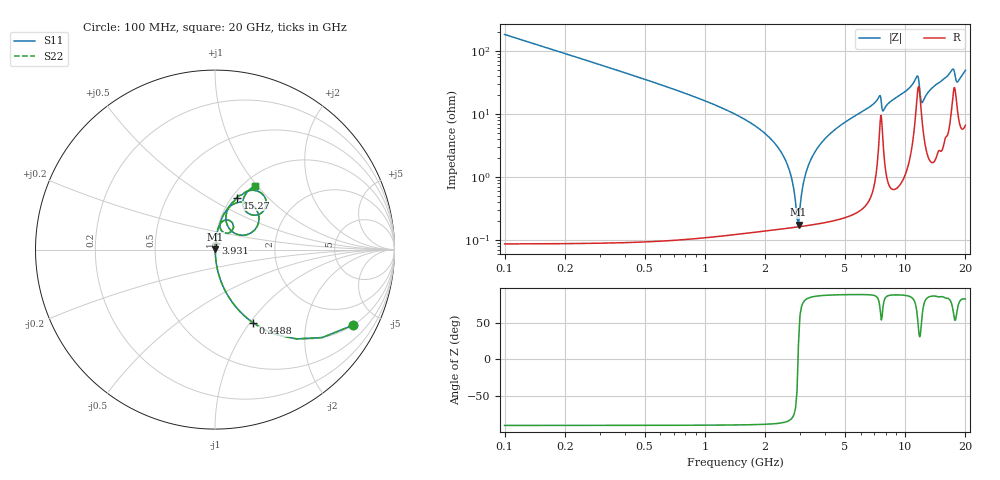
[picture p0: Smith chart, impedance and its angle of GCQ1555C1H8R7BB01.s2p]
!Murata Part Number: GCQ1555C1H8R7BB01
!These Parameters are Measured in Series Mode Connection
!Data Generated on Mar 13, 2026
!  o--ll--o
!Port1  Port2
!  o------o
!Operation Temp=25[degC], DC Bias Voltage=0[V]
!Freq. Start=100[MHz] Stop=20[GHz] 401[Steps]
# Hz S RI R 50
!Freq.(Hz) S11(Real) S11(Imag) S21(Real) S21(Imag) S12(Real) S12(Imag) S22(Real) S22(Imag)
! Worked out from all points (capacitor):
!   401 points, 100 MHz to 20 GHz, reference 50 ohm
!   read as one part in series: C = 8.7 pF near 199.5 MHz
!   lowest |Z| = 174 mohm at 2.936 GHz (marker M1)
!   series resonance near 2.92 GHz, so ESL is about 340 pH
!   S11 on the Smith chart (normalised r, x): 100 MHz: 1.00, -3.65; 348.8 MHz: 1.00, -1.03; 3.931 GHz: 1.00, +0.08; 15.27 GHz: 1.05, +0.68; 20 GHz: 1.13, +0.98
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1e8  0.7694 -0.421  0.2306 0.421  0.2306 0.421  0.7694 -0.421
3.4875e8  0.2113 -0.4074  0.7887 0.4074  0.7887 0.4074  0.2113 -0.4074
8.4625e8  0.0386 -0.1902  0.9614 0.1902  0.9614 0.1902  0.0386 -0.1902
2.33875e9  0.00225 -0.0281  0.9977 0.0281  0.9977 0.0281  0.00225 -0.0281
2.63725e9  0.0017 -0.0128  0.9983 0.0128  0.9983 0.0128  0.0017 -0.0128
2.83625e9  0.00159 -0.00368  0.9984 0.00368  0.9984 0.00368  0.00159 -0.00368
2.93575e9  0.0016 0.000665  0.9984 -0.000665  0.9984 -0.000665  0.0016 0.000665
3.1845e9  0.00178 0.0109  0.9982 -0.0109  0.9982 -0.0109  0.00178 0.0109
3.43325e9  0.00215 0.0206  0.9979 -0.0206  0.9979 -0.0206  0.00215 0.0206
3.93075e9  0.00333 0.0383  0.9967 -0.0383  0.9967 -0.0383  0.00333 0.0383
6.7665e9  0.0224 0.1306  0.9776 -0.1306  0.9776 -0.1306  0.0224 0.1306
7.463e9  0.0816 0.1621  0.9184 -0.1621  0.9184 -0.1621  0.0816 0.1621
7.81125e9  0.0367 0.1048  0.9633 -0.1048  0.9633 -0.1048  0.0367 0.1048
1.005e10  0.0593 0.2131  0.9407 -0.2131  0.9407 -0.2131  0.0593 0.2131
1.149275e10  0.2292 0.2244  0.7708 -0.2244  0.7708 -0.2244  0.2292 0.2244
1.21395e10  0.0877 0.1075  0.9123 -0.1075  0.9123 -0.1075  0.0877 0.1075
1.338325e10  0.07 0.2215  0.93 -0.2215  0.93 -0.2215  0.07 0.2215
1.527375e10  0.1212 0.2898  0.8788 -0.2898  0.8788 -0.2898  0.1212 0.2898
1.67165e10  0.2006 0.3303  0.7994 -0.3303  0.7994 -0.3303  0.2006 0.3303
1.746275e10  0.286 0.2593  0.714 -0.2593  0.714 -0.2593  0.286 0.2593
1.81095e10  0.178 0.2075  0.822 -0.2075  0.822 -0.2075  0.178 0.2075
2e10  0.2252 0.3558  0.7748 -0.3558  0.7748 -0.3558  0.2252 0.3558
